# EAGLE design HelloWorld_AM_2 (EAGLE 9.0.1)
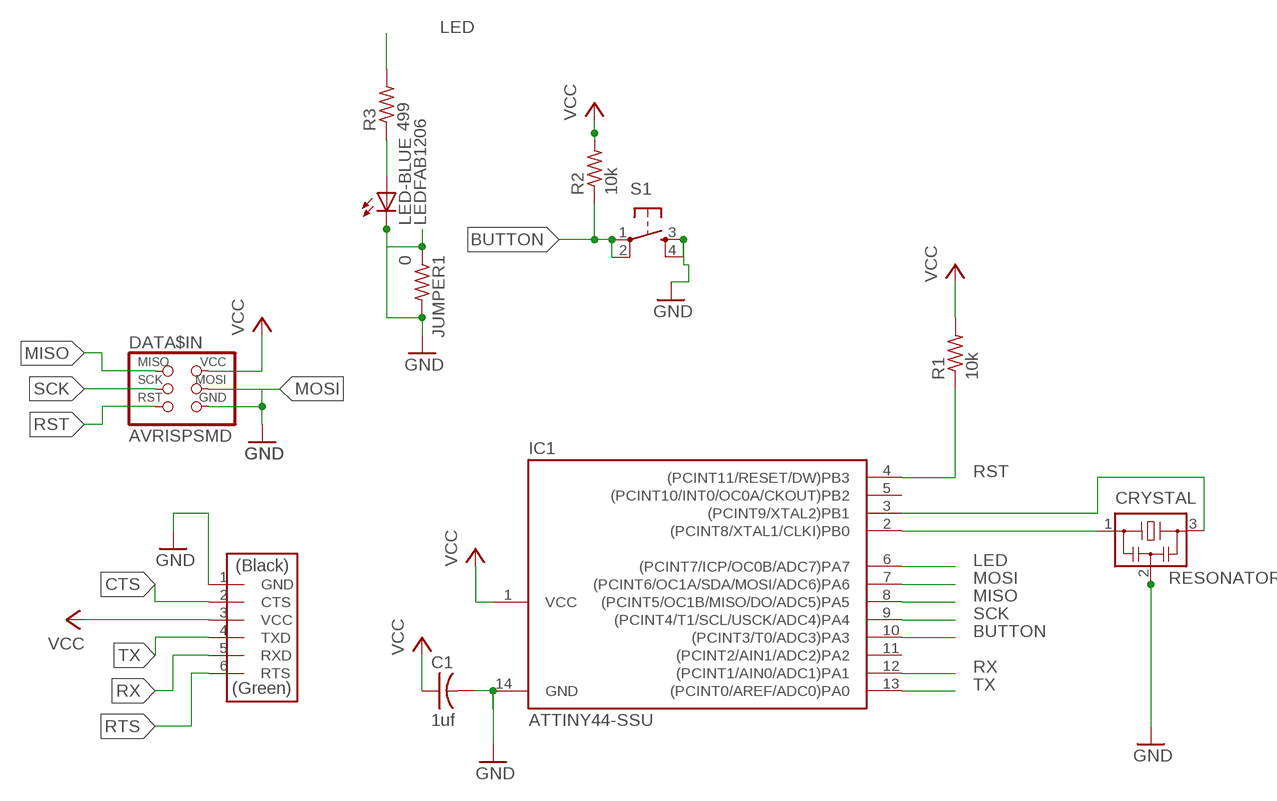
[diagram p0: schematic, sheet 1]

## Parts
C1  1uf  CAP-US1206FAB  [C1206FAB]
CRYSTAL  RESONATOR  [EFOBM]
DATA$IN  AVRISPSMD  [2X03SMD]
DATA$OUT  FTDI-SMD-HEADER  [1X06SMD]
IC1  ATTINY44-SSU  [SOIC14]
JUMPER1  0  RES-US1206FAB  [R1206FAB]
LED-BLUE  LEDFAB1206  [LED1206FAB]
R1  10k  RES-US1206FAB  [R1206FAB]
R2  10k  RES-US1206FAB  [R1206FAB]
R3  499  RES-US1206FAB  [R1206FAB]
S1  6MM_SWITCH6MM_SWITCH  [6MM_SWITCH]

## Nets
BUTTON: IC1.10((PCINT3/T0/ADC3)PA3) R2.1 S1.1(P) S1.2(P1)
CTS: DATA$OUT.2(CTS)
GND: C1.2 CRYSTAL.2 DATA$IN.6(GND) DATA$OUT.1(GND) IC1.14(GND) JUMPER1.1 JUMPER1.2 LED-BLUE.2(C) S1.3(S) S1.4(S1)
LED: IC1.6((PCINT7/ICP/OC0B/ADC7)PA7) R3.2
MISO: DATA$IN.1(MISO) IC1.8((PCINT5/OC1B/MISO/DO/ADC5)PA5)
MOSI: DATA$IN.4(MOSI) IC1.7((PCINT6/OC1A/SDA/MOSI/ADC6)PA6)
N$1: CRYSTAL.1 IC1.2((PCINT8/XTAL1/CLKI)PB0)
N$3: LED-BLUE.1(A) R3.1
N$7: CRYSTAL.3 IC1.3((PCINT9/XTAL2)PB1)
RST: DATA$IN.5(RST) IC1.4((PCINT11/RESET/DW)PB3) R1.1
RTS: DATA$OUT.6(RTS)
RX: DATA$OUT.5(RXD) IC1.12((PCINT1/AIN0/ADC1)PA1)
SCK: DATA$IN.3(SCK) IC1.9((PCINT4/T1/SCL/USCK/ADC4)PA4)
TX: DATA$OUT.4(TXD) IC1.13((PCINT0/AREF/ADC0)PA0)
VCC: C1.1 DATA$IN.2(VCC) DATA$OUT.3(VCC) IC1.1(VCC) R1.2 R2.2
Unconnected: IC1.5((PCINT10/INT0/OC0A/CKOUT)PB2) IC1.11((PCINT2/AIN1/ADC2)PA2)

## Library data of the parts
C1 = fab:CAP-US
CRYSTAL = fab:RESONATOR
DATA$IN = fab:AVRISP
DATA$OUT = fab:FTDI-SMD-HEADER
IC1 = fab:ATTINY44
JUMPER1 R1-R3 = fab:RES-US: Resistor (US Symbol)
LED-BLUE = fab:LED: LED
S1 = fab:6MM_SWITCH: OMRON SWITCH

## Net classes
0 default: width 0.254 mm, drill 0.508 mm, clearance 0.305 mm

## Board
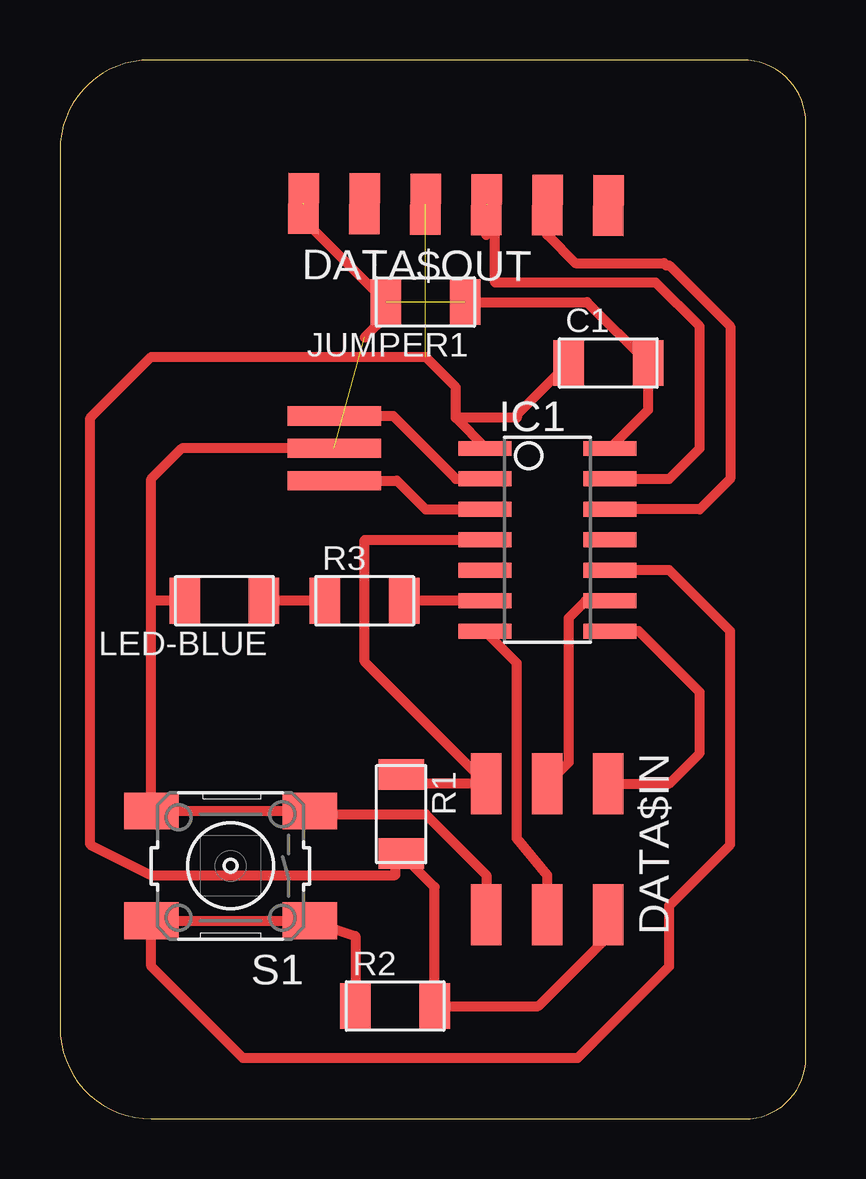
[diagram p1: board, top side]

Size 31.09 x 44.12 mm. Coordinates in mm from the lower left corner, seen from the top.
Outline: 31.09,2.54 31.09,41.49 arc90 28.46,44.12 3.75,44.12 arc90 0,40.37 0,3.81 arc90 3.81,0 28.55,0 arc90 31.09,2.54
Copper layers (1*16): Top 0.035mm / dielectric 1.5mm / Bottom 0.035mm
Design rules "default *": minimum track width 16mil, minimum drill 0.35mm, track to track 16mil, track to pad 16mil, pad to pad 16mil, via to via 16mil, smd to smd 16mil, copper to edge 16mil, drill to drill 16mil, minimum pad ring 10mil, minimum via ring 8mil, stop-mask expansion 4mil, vias tented up to drill 0mil, thermal gap 10mil

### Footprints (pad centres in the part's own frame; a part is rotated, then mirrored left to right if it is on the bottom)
C1206FAB = smd 1.27 x 1.905: 1 -1.651,0; 2 1.651,0
EFOBM = smd 0.8 x 3.9: 1 -1.35,0; 2 0,0; 3 1.35,0
2X03SMD = smd 2.54 x 1.27: 1 -2.54,2.54; 2 2.92,2.54; 3 -2.54,0; 4 2.92,0; 5 -2.54,-2.54; 6 2.92,-2.54
1X06SMD = smd 2.54 x 1.27: 1 0,6.35; 2 0,3.81; 3 0,1.27; 4 0,-1.27; 5 0,-3.81; 6 0,-6.35
SOIC14 = smd 0.61 x 2.21: 1 -3.81,-2.603; 2 -2.54,-2.603; 3 -1.27,-2.603; 4 0,-2.603; 5 1.27,-2.603; 6 2.54,-2.603; 7 3.81,-2.603; 8 3.81,2.603; 9 2.54,2.603; 10 1.27,2.603; 11 0,2.603; 12 -1.27,2.603; 13 -2.54,2.603; 14 -3.81,2.603
R1206FAB = smd 1.27 x 1.905: 1 -1.651,0; 2 1.651,0
LED1206FAB = smd 1.27 x 1.905: 1 -1.651,0; 2 1.651,0
6MM_SWITCH = smd 2.286 x 1.524: 1 -3.302,2.286; 2 3.302,2.286; 3 -3.302,-2.286; 4 3.302,-2.286

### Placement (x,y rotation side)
C1  22.86,31.5 0 top
CRYSTAL  11.43,27.94 270 top
DATA$IN  20.32,11.43 270 top
DATA$OUT  16.51,38.1 89.6 top
IC1  20.32,24.13 270 top
JUMPER1  15.24,34.04 180 top
LED-BLUE  6.86,21.59 180 top
R1  14.22,12.7 270 top
R2  13.97,4.7 0 top
R3  12.7,21.59 0 top
S1  7.11,10.54 180 top

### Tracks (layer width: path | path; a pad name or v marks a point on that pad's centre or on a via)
BUTTON
  Top 0.406: IC1.10 25.4,22.86 27.94,20.32 27.94,11.43 25.4,8.89 25.4,6.35 21.59,2.54 7.62,2.54 3.81,6.35 S1.2 S1.1 12.32,7.62 R2.1
GND  (3 unrouted)
  Top 0.406: CRYSTAL.2 5.08,27.94 3.81,26.67 3.81,21.59 | IC1.14 24.51,29.53 C1.2 21.97,34.04 JUMPER1.1 | DATA$IN.6 17.78,10.16 15.24,12.7 10.54,12.7 S1.3 S1.4 3.81,21.59 | LED-BLUE.2 3.81,21.59 | 10.03,38.1 10.16,38.1 10.16,37.47 JUMPER1.2 13.59,33.45 12.7,32.56
LED
  Top 0.406: IC1.6 R3.2
MISO
  Top 0.406: DATA$IN.1 25.4,13.97 26.67,15.24 26.67,17.78 24.13,20.32 IC1.8
MOSI
  Top 0.406: 17.78,20.26 IC1.7 19.05,18.99 19.05,11.68 20.32,10.16 DATA$IN.4
N$1
  Top 0.406: CRYSTAL.1 13.89,29.29 16.51,26.67 IC1.2
N$3
  Top 0.406: R3.1 LED-BLUE.1
N$7
  Top 0.406: CRYSTAL.3 14.05,26.59 15.24,25.4 IC1.3
RST
  Top 0.406: R1.1 14.61,13.97 DATA$IN.5 12.7,19.05 12.7,24.13 IC1.4
RX
  Top 0.406: IC1.12 26.67,25.4 27.94,26.67 27.94,33.02 25.4,35.56 25.28,35.56 25.18,35.66 21.49,35.66 20.32,36.83 DATA$OUT.5
SCK
  Top 0.406: DATA$IN.3 21.21,14.86 21.21,20.88 21.92,21.59 IC1.9
TX  (1 unrouted)
  Top 0.406: 17.78,36.83 DATA$OUT.4 18.14,37.74 18.14,34.85 24.84,34.85 26.67,33.02 26.67,30.48 26.67,27.94 25.4,26.67 IC1.13
VCC  (1 unrouted)
  Top 0.406: 21.21,31.43 C1.1 19.05,29.34 19.05,29.21 16.51,29.21 | 16.51,29.21 17.75,27.97 IC1.1 | DATA$IN.2 22.86,7.62 19.94,4.7 R2.2 15.62,9.65 R1.2 13.97,10.79 13.97,10.16 3.81,10.16 1.27,11.43 1.27,29.21 3.81,31.75 15.24,31.75 16.51,30.48 16.51,29.21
